| This Model is valid for Automotive grade 2 Temperature Range -40C<=Tc<=105C
| Valid for LPDDR4-4266 operation
| Part Number   VDD/VDDQ   Package   Architecture
| SCE11U32322EF-04ZA2   1.1 +0.07/-0.04  FBGA   1G   bit x 32 (200b,DDP,10x14.5x1.1)
| SCE11U16320EF-04ZA2   1.1 +0.07/-0.04  FBGA   512M bit x 32 (200b,SDP,10x14.5x1.1)
[IBIS Ver]  5.0
[File Name] usesnxx32fa2.ibs
[Date]   05/20/2025
[File Rev]  1.0
[Source] Simulation of a silicon level SPICE model
[Notes]  IBIS Characteristics for I/O Buffer
  IBIS Model Revision History: Rev 2.0:
  2026-03-27 - IBIS model file PN number change
[Disclaimer]  The IBIS models are for modeling purpose only and are subject to change without any notice. UniIC is not
  responsible for any problems the models may cause.
[Copyright] Copyright 2025 UniIC Semiconductors Corp. All rights reserved
|   Component SCE11U32322EF-04ZA2
[Component] SCE11U32322EF-04ZA2
[Manufacturer] UniIC Semiconductors Corp.
[Package]
|   typ   min   max
R_pkg   1104.5m   650.50m   1552.0m
L_pkg   2.074nH   1.252nH   2.895nH
C_pkg   0.931pF   0.710pF   1.151pF
[Pin] signal_name  model_name   R_pin   L_pin   C_pin
A1   DNU   NC
A2   DNU   NC
A3   VSS   GND
A4   VDD2   POWER
A5   ZQ0   NC
A8   NC   NC
A9   VDD2   POWER
A10   VSS   GND
A11   DNU   NC
A12   DNU   NC
B1   DNU   NC
B2   DQ0_A   DQ   847.00m   1.698nH   0.760pF
B3   VDDQ   POWER
B4   DQ7_A   DQ   926.00m   1.813nH   0.812pF
B5   VDDQ   POWER
B8   VDDQ   POWER
B9   DQ15_A   DQ   770.00m   1.540nH   0.721pF
B10   VDDQ   POWER
B11   DQ8_A   DQ   887.00m   1.780nH   0.770pF
B12   DNU   NC
C1   VSS   GND
C2   DQ1_A   DQ   875.00m   1.700nH   0.768pF
C3   DMI0_A   DQ   814.00m   1.560nH   0.737pF
C4   DQ6_A   DQ   807.82m   1.550nH   0.748pF
C5   VSS   GND
C8   VSS   GND
C9   DQ14_A   DQ   734.60m   1.445nH   0.710pF
C10   DMI1_A   DQ   797.00m   1.548nH   0.747pF
C11   DQ9_A   DQ   850.56m   1.652nH   0.773pF
C12   VSS   GND
D1   VDDQ   POWER
D2   VSS   GND
D3   DQS0_t_A   DQS   876.90m   1.604nH   0.763pF
D4   VSS   GND
D5   VDDQ   POWER
D8   VDDQ   POWER
D9   VSS   GND
D10   DQS1_t_A   DQS   887.69m   1.639nH   0.761pF
D11   VSS   GND
D12   VDDQ   POWER
E1   VSS   GND
E2   DQ2_A   DQ   762.89m   1.467nH   0.748pF
E3   DQS0_c_A   DQS   844.00m   1.542nH   0.754pF
E4   DQ5_A   DQ   703.98m   1.301nH   0.737pF
E5   VSS   GND
E8   VSS   GND
E9   DQ13_A   DQ   773.00m   1.436nH   0.777pF
E10   DQS1_c_A   DQS   883.30m   1.623nH   0.758pF
E11   DQ10_A   DQ   765.46m   1.468nH   0.760pF
E12   VSS   GND
F1   VDD1   POWER
F2   DQ3_A   DQ   779.40m   1.504nH   0.756pF
F3   VDDQ   POWER
F4   DQ4_A   DQ   716.48m   1.324nH   0.756pF
F5   VDD2   POWER
F8   VDD2   POWER
F9   DQ12_A   DQ   662.23m   1.252nH   0.714pF
F10   VDDQ   POWER
F11   DQ11_A   DQ   774.23m   1.506nH   0.768pF
F12   VDD1   POWER
G1   VSS   GND
G2   ODT_CA_A   ODTCA_INPUT   1136.0m   2.180nH   0.892pF
G3   VSS   GND
G4   VDD1   POWER
G5   VSS   GND
G8   VSS   GND
G9   VDD1   POWER
G10   VSS   GND
G11   NC   NC
G12   VSS   GND
H1   VDD2   POWER
H2   CA0_A   CA_INPUT   1398.8m   2.593nH   1.130pF
H3   CS1_A   CS_INPUT
H4   CS0_A   CS_INPUT
H5   VDD2   POWER
H8   VDD2   POWER
H9   CA2_A   CA_INPUT   1397.0m   2.554nH   1.150pF
H10   CA3_A   CA_INPUT   1148.0m   2.598nH   1.143pF
H11   CA4_A   CA_INPUT   1148.0m   2.709nH   1.153pF
H12   VDD2   POWER
J1   VSS   GND
J2   CA1_A   CA_INPUT   1453.0m   2.712nH   1.151pF
J3   VSS   GND
J4   CKE0_A   CKE_INPUT
J5   CKE1_A   CKE_INPUT
J8   CK_t_A   CLK_INPUT   1469.0m   2.704nH   1.078pF
J9   CK_c_A   CLK_INPUT   1486.0m   2.711nH   1.095pF
J10   VSS   GND
J11   CA5_A   CA_INPUT   1552.0m   2.895nH   1.206pF
J12   VSS   GND
K1   VDD2   POWER
K2   VSS   GND
K3   VDD2   POWER
K4   VSS   GND
K5   NC   NC
K8   NC   NC
K9   VSS   GND
K10   VDD2   POWER
K11   VSS   GND
K12   VDD2   POWER
N1   VDD2   POWER
N2   VSS   GND
N3   VDD2   POWER
N4   VSS   GND
N5   NC   NC
N8   NC   NC
N9   VSS   GND
N10   VDD2   POWER
N11   VSS   GND
N12   VDD2   POWER
P1   VSS   GND
P2   CA1_B   CA_INPUT   1442.0m   2.680nH   1.156pF
P3   VSS   GND
P4   CKE0_B   CKE_INPUT
P5   CKE1_B   CKE_INPUT
P8   CK_t_B   CLK_INPUT   1474.0m   2.686nH   1.065pF
P9   CK_c_B   CLK_INPUT   1481.0m   2.692nH   1.076pF
P10   VSS   GND
P11   CA5_B   CA_INPUT   1535.0m   2.859nH   1.204pF
P12   VSS   GND
R1   VDD2   POWER
R2   CA0_B   CA_INPUT   1435.0m   2.641nH   1.133pF
R3   CS1_B   CS_INPUT
R4   CS0_B   CS_INPUT
R5   VDD2   POWER
R8   VDD2   POWER
R9   CA2_B   CA_INPUT   1374.0m   2.528nH   1.124pF
R10   CA3_B   CA_INPUT   1373.0m   2.527nH   1.125pF
R11   CA4_B   CA_INPUT   1463.0m   2.722nH   1.149pF
R12   VDD2   POWER
T1   VSS   GND
T2   ODT_CA_B   ODTCA_INPUT   1146.0m   2.205nH   0.900pF
T3   VSS   GND
T4   VDD1   POWER
T5   VSS   GND
T8   VSS   GND
T9   VDD1   POWER
T10   VSS   GND
T11   RESET_n   NC
T12   VSS   GND
U1   VDD1   POWER
U2   DQ3_B   DQ   804.00m   1.559nH   0.763pF
U3   VDDQ   POWER
U4   DQ4_B   DQ   687.00m   1.284nH   0.716pF
U5   VDD2   POWER
U8   VDD2   POWER
U9   DQ12_B   DQ   672.30m   1.262nH   0.724pF
U10   VDDQ   POWER
U11   DQ11_B   DQ   777.17m   1.513nH   0.758pF
U12   VDD1   POWER
V1   VSS   GND
V2   DQ2_B   DQ   797.40m   1.539nH   0.769pF
V3   DQS0_c_B   DQS   861.50m   1.603nH   0.741pF
V4   DQ5_B   DQ   650.50m   1.233nH   0.701pF
V5   VSS   GND
V8   VSS   GND
V9   DQ13_B   DQ   648.00m   1.227nH   0.706pF
V10   DQS1_c_B   DQS   841.00m   1.538nH   0.744pF
V11   DQ10_B   DQ   771.40m   1.488nH   0.759pF
V12   VSS   GND
W1   VDDQ   POWER
W2   VSS   GND
W3   DQS0_t_B   DQS   839.00m   1.577nH   0.740pF
W4   VSS   GND
W5   VDDQ   POWER
W8   VDDQ   POWER
W9   VSS   GND
W10   DQS1_t_B   DQS   841.00m   1.547nH   0.733pF
W11   VSS   GND
W12   VDDQ   POWER
Y1   VSS   GND
Y2   DQ1_B   DQ   911.00m   1.744nH   0.787pF
Y3   DMI0_B   DQ   814.40m   1.570nH   0.726pF
Y4   DQ6_B   DQ   768.00m   1.499nH   0.718pF
Y5   VSS   GND
Y8   VSS   GND
Y9   DQ14_B   DQ   804.26m   1.578nH   0.754pF
Y10   DMI1_B   DQ   823.20m   1.578nH   0.761pF
Y11   DQ9_B   DQ   877.50m   1.697nH   0.780pF
Y12   VSS   GND
AA1   DNU   NC
AA2   DQ0_B   DQ   830.50m   1.680nH   0.752pF
AA3   VDDQ   POWER
AA4   DQ7_B   DQ   782.00m   1.584nH   0.730pF
AA5   VDDQ   POWER
AA8   VDDQ   POWER
AA9   DQ15_B   DQ   855.00m   1.687nH   0.761pF
AA10  VDDQ   POWER
AA11  DQ8_B   DQ   834.70m   1.680nH   0.751pF
AA12  DNU   NC
AB1   DNU   NC
AB2   DNU   NC
AB3   VSS   GND
AB4   VDD2   POWER
AB5   VSS   GND
AB8   VSS   GND
AB9   VDD2   POWER
AB10  VSS   GND
AB11  DNU   NC
AB12  DNU   NC
[Diff Pin]  inv_pin  vdiff   tdelay_typ   tdelay_min   tdelay_max
D3   E3   0.120V   0.000s   NA   NA
W3   V3   0.120V   0.000s   NA   NA
D10   E10   0.120V   0.000s   NA   NA
W10   V10   0.120V   0.000s   NA   NA
J8   J9   0.145V   0.000s   NA   NA
P8   P9   0.145V   0.000s   NA   NA
|   Component SCE11U16320EF-04ZA2
[Component] SCE11U16320EF-04ZA2
[Manufacturer] UniIC Semiconductors Corp.
[Package]
|   typ   min   max
R_pkg   1781.0m   683.00m   3340.0m
L_pkg   3.313nH   1.222nH   6.060nH
C_pkg   1.150pF   0.604pF   2.030pF
[Pin] signal_name  model_name   R_pin   L_pin   C_pin
A1   DNU   NC
A2   DNU   NC
A3   VSS   GND
A4   VDD2   POWER
A5   ZQ0   NC
A8   NC   NC
A9   VDD2   POWER
A10   VSS   GND
A11   DNU   NC
A12   DNU   NC
B1   DNU   NC
B2   DQ0_A   DQ   847.00m   1.698nH   0.760pF
B3   VDDQ   POWER
B4   DQ7_A   DQ   926.00m   1.813nH   0.812pF
B5   VDDQ   POWER
B8   VDDQ   POWER
B9   DQ15_A   DQ   770.00m   1.540nH   0.721pF
B10   VDDQ   POWER
B11   DQ8_A   DQ   887.00m   1.780nH   0.770pF
B12   DNU   NC
C1   VSS   GND
C2   DQ1_A   DQ   875.00m   1.700nH   0.768pF
C3   DMI0_A   DQ   814.00m   1.560nH   0.737pF
C4   DQ6_A   DQ   807.82m   1.550nH   0.748pF
C5   VSS   GND
C8   VSS   GND
C9   DQ14_A   DQ   734.60m   1.445nH   0.710pF
C10   DMI1_A   DQ   797.00m   1.548nH   0.747pF
C11   DQ9_A   DQ   850.56m   1.652nH   0.773pF
C12   VSS   GND
D1   VDDQ   POWER
D2   VSS   GND
D3   DQS0_t_A   DQS   876.90m   1.604nH   0.763pF
D4   VSS   GND
D5   VDDQ   POWER
D8   VDDQ   POWER
D9   VSS   GND
D10   DQS1_t_A   DQS   887.69m   1.639nH   0.761pF
D11   VSS   GND
D12   VDDQ   POWER
E1   VSS   GND
E2   DQ2_A   DQ   762.89m   1.467nH   0.748pF
E3   DQS0_c_A   DQS   844.00m   1.542nH   0.754pF
E4   DQ5_A   DQ   703.98m   1.301nH   0.737pF
E5   VSS   GND
E8   VSS   GND
E9   DQ13_A   DQ   773.00m   1.436nH   0.777pF
E10   DQS1_c_A   DQS   883.30m   1.623nH   0.758pF
E11   DQ10_A   DQ   765.46m   1.468nH   0.760pF
E12   VSS   GND
F1   VDD1   POWER
F2   DQ3_A   DQ   779.40m   1.504nH   0.756pF
F3   VDDQ   POWER
F4   DQ4_A   DQ   716.48m   1.324nH   0.756pF
F5   VDD2   POWER
F8   VDD2   POWER
F9   DQ12_A   DQ   662.23m   1.252nH   0.714pF
F10   VDDQ   POWER
F11   DQ11_A   DQ   774.23m   1.506nH   0.768pF
F12   VDD1   POWER
G1   VSS   GND
G2   ODT_CA_A   ODTCA_INPUT   1136.0m   2.180nH   0.892pF
G3   VSS   GND
G4   VDD1   POWER
G5   VSS   GND
G8   VSS   GND
G9   VDD1   POWER
G10   VSS   GND
G11   NC   NC
G12   VSS   GND
H1   VDD2   POWER
H2   CA0_A   CA_INPUT   1398.8m   2.593nH   1.13pF
H3   NC   NC
H4   CS0_A   CS_INPUT
H5   VDD2   POWER
H8   VDD2   POWER
H9   CA2_A   CA_INPUT   1397.0m   2.554nH   1.150pF
H10   CA3_A   CA_INPUT   1148.0m   2.598nH   1.143pF
H11   CA4_A   CA_INPUT   1148.0m   2.709nH   1.153pF
H12   VDD2   POWER
J1   VSS   GND
J2   CA1_A   CA_INPUT   1453.0m   2.712nH   1.151pF
J3   VSS   GND
J4   CKE0_A   CKE_INPUT
J5   NC   NC
J8   CK_t_A   CLK_INPUT   1469.0m   2.704nH   1.078pF
J9   CK_c_A   CLK_INPUT   1486.0m   2.711nH   1.095pF
J10   VSS   GND
J11   CA5_A   CA_INPUT   1552.0m   2.895nH   1.206pF
J12   VSS   GND
K1   VDD2   POWER
K2   VSS   GND
K3   VDD2   POWER
K4   VSS   GND
K5   NC   NC
K8   NC   NC
K9   VSS   GND
K10   VDD2   POWER
K11   VSS   GND
K12   VDD2   POWER
N1   VDD2   POWER
N2   VSS   GND
N3   VDD2   POWER
N4   VSS   GND
N5   NC   NC
N8   NC   NC
N9   VSS   GND
N10   VDD2   POWER
N11   VSS   GND
N12   VDD2   POWER
P1   VSS   GND
P2   CA1_B   CA_INPUT   1442.0m   2.680nH   1.156pF
P3   VSS   GND
P4   CKE0_B   CKE_INPUT
P5   NC   NC
P8   CK_t_B   CLK_INPUT   1474.0m   2.686nH   1.065pF
P9   CK_c_B   CLK_INPUT   1481.0m   2.692nH   1.076pF
P10   VSS   GND
P11   CA5_B   CA_INPUT   1535.0m   2.859nH   1.204pF
P12   VSS   GND
R1   VDD2   POWER
R2   CA0_B   CA_INPUT   1435.0m   2.641nH   1.133pF
R3   NC   NC
R4   CS0_B   CS_INPUT
R5   VDD2   POWER
R8   VDD2   POWER
R9   CA2_B   CA_INPUT   1374.0m   2.528nH   1.124pF
R10   CA3_B   CA_INPUT   1373.0m   2.527nH   1.125pF
R11   CA4_B   CA_INPUT   1463.0m   2.722nH   1.149pF
R12   VDD2   POWER
T1   VSS   GND
T2   ODT_CA_B   ODTCA_INPUT   1146.0m   2.205nH   0.900pF
T3   VSS   GND
T4   VDD1   POWER
T5   VSS   GND
T8   VSS   GND
T9   VDD1   POWER
T10   VSS   GND
T11   RESET_n   NC
T12   VSS   GND
U1   VDD1   POWER
U2   DQ3_B   DQ   804.00m   1.559nH   0.763pF
U3   VDDQ   POWER
U4   DQ4_B   DQ   687.00m   1.284nH   0.716pF
U5   VDD2   POWER
U8   VDD2   POWER
U9   DQ12_B   DQ   672.30m   1.262nH   0.724pF
U10   VDDQ   POWER
U11   DQ11_B   DQ   777.17m   1.513nH   0.758pF
U12   VDD1   POWER
V1   VSS   GND
V2   DQ2_B   DQ   797.40m   1.539nH   0.769pF
V3   DQS0_c_B   DQS   861.50m   1.603nH   0.741pF
V4   DQ5_B   DQ   650.50m   1.233nH   0.701pF
V5   VSS   GND
V8   VSS   GND
V9   DQ13_B   DQ   648.00m   1.227nH   0.706pF
V10   DQS1_c_B   DQS   841.00m   1.538nH   0.744pF
V11   DQ10_B   DQ   771.40m   1.488nH   0.759pF
V12   VSS   GND
W1   VDDQ   POWER
W2   VSS   GND
W3   DQS0_t_B   DQS   839.00m   1.577nH   0.740pF
W4   VSS   GND
W5   VDDQ   POWER
W8   VDDQ   POWER
W9   VSS   GND
W10   DQS1_t_B   DQS   841.00m   1.547nH   0.733pF
W11   VSS   GND
W12   VDDQ   POWER
Y1   VSS   GND
Y2   DQ1_B   DQ   911.00m   1.744nH   0.787pF
Y3   DMI0_B   DQ   814.40m   1.570nH   0.726pF
Y4   DQ6_B   DQ   768.00m   1.499nH   0.718pF
Y5   VSS   GND
Y8   VSS   GND
Y9   DQ14_B   DQ   804.26m   1.578nH   0.754pF
Y10   DMI1_B   DQ   823.20m   1.578nH   0.761pF
Y11   DQ9_B   DQ   877.50m   1.697nH   0.780pF
Y12   VSS   GND
AA1   DNU   NC
AA2   DQ0_B   DQ   830.50m   1.680nH   0.752pF
AA3   VDDQ   POWER
AA4   DQ7_B   DQ   782.00m   1.584nH   0.730pF
AA5   VDDQ   POWER
AA8   VDDQ   POWER
AA9   DQ15_B   DQ   855.00m   1.687nH   0.761pF
AA10  VDDQ   POWER
AA11  DQ8_B   DQ   834.70m   1.680nH   0.751pF
AA12  DNU   NC
AB1   DNU   NC
AB2   DNU   NC
AB3   VSS   GND
AB4   VDD2   POWER
AB5   VSS   GND
AB8   VSS   GND
AB9   VDD2   POWER
AB10  VSS   GND
AB11  DNU   NC
AB12  DNU   NC
[Diff Pin]  inv_pin  vdiff   tdelay_typ   tdelay_min   tdelay_max
D3   E3   0.120V   0.000s   NA   NA
W3   V3   0.120V   0.000s   NA   NA
D10   E10   0.120V   0.000s   NA   NA
W10   V10   0.120V   0.000s   NA   NA
J8   J9   0.145V   0.000s   NA   NA
P8   P9   0.145V   0.000s   NA   NA
|   Model Selector
[Model Selector] DQ
| Data I/O models
DQ_PD40_SOC-ODT40_VOH30_4266   40 Ohm Pulldown, 40 Ohm System ODT Setting, VOH=VDDQ/3.0, 3200-4266Mbps
DQ_PD40_SOC-ODT48_VOH30_4266   40 Ohm Pulldown, 48 Ohm System ODT Setting, VOH=VDDQ/3.0, 3200-4266Mbps
DQ_PD40_SOC-ODT60_VOH30_4266   40 Ohm Pulldown, 60 Ohm System ODT Setting, VOH=VDDQ/3.0, 3200-4266Mbps
DQ_PD40_SOC-ODT80_VOH30_4266   40 Ohm Pulldown, 80 Ohm System ODT Setting, VOH=VDDQ/3.0, 3200-4266Mbps
DQ_PD40_SOC-ODT120_VOH30_4266   40 Ohm Pulldown, 120 Ohm System ODT Setting, VOH=VDDQ/3.0, 3200-4266Mbps
DQ_PD40_SOC-ODT240_VOH30_4266   40 Ohm Pulldown, 240 Ohm System ODT Setting, VOH=VDDQ/3.0, 3200-4266Mbps
DQ_PD40_SOC-ODTDIS_VOH30_4266   40 Ohm Pulldown, SOC ODT disabled setting, VOH=VDDQ/3.0 cal. point, 3200-4266Mbps
DQ_PD40_SOC-ODT80_VOH25_4266   40 Ohm Pulldown, 80 Ohm System ODT Setting, VOH=VDDQ/2.5, 3200-4266Mbps
DQ_PD40_SOC-ODT120_VOH25_4266   40 Ohm Pulldown, 120 Ohm System ODT Setting, VOH=VDDQ/2.5, 3200-4266Mbps
DQ_PD40_SOC-ODT240_VOH25_4266   40 Ohm Pulldown, 240 Ohm System ODT Setting, VOH=VDDQ/2.5, 3200-4266Mbps
DQ_PD40_SOC-ODTDIS_VOH25_4266   40 Ohm Pulldown, SOC ODT disabled setting, VOH=VDDQ/2.5 cal. point, 3200-4266Mbps
DQ_PD48_SOC-ODT40_VOH30_4266   48 Ohm Pulldown, 40 Ohm System ODT Setting, VOH=VDDQ/3.0, 3200-4266Mbps
DQ_PD48_SOC-ODT48_VOH30_4266   48 Ohm Pulldown, 48 Ohm System ODT Setting, VOH=VDDQ/3.0, 3200-4266Mbps
DQ_PD48_SOC-ODT60_VOH30_4266   48 Ohm Pulldown, 60 Ohm System ODT Setting, VOH=VDDQ/3.0, 3200-4266Mbps
DQ_PD48_SOC-ODT80_VOH30_4266   48 Ohm Pulldown, 80 Ohm System ODT Setting, VOH=VDDQ/3.0, 3200-4266Mbps
DQ_PD48_SOC-ODT120_VOH30_4266   48 Ohm Pulldown, 120 Ohm System ODT Setting, VOH=VDDQ/3.0, 3200-4266Mbps
DQ_PD48_SOC-ODT240_VOH30_4266   48 Ohm Pulldown, 240 Ohm System ODT Setting, VOH=VDDQ/3.0, 3200-4266Mbps
DQ_PD48_SOC-ODTDIS_VOH30_4266   48 Ohm Pulldown, SOC ODT disabled setting, VOH=VDDQ/3.0 cal. point, 3200-4266Mbps
DQ_PD48_SOC-ODT80_VOH25_4266   48 Ohm Pulldown, 80 Ohm System ODT Setting, VOH=VDDQ/2.5, 3200-4266Mbps
DQ_PD48_SOC-ODT120_VOH25_4266   48 Ohm Pulldown, 120 Ohm System ODT Setting, VOH=VDDQ/2.5, 3200-4266Mbps
DQ_PD48_SOC-ODT240_VOH25_4266   48 Ohm Pulldown, 240 Ohm System ODT Setting, VOH=VDDQ/2.5, 3200-4266Mbps
DQ_PD48_SOC-ODTDIS_VOH25_4266   48 Ohm Pulldown, SOC ODT disabled setting, VOH=VDDQ/2.5 cal. point, 3200-4266Mbps
DQ_PD60_SOC-ODT40_VOH30_4266   60 Ohm Pulldown, 40 Ohm System ODT Setting, VOH=VDDQ/3.0, 3200-4266Mbps
DQ_PD60_SOC-ODT48_VOH30_4266   60 Ohm Pulldown, 48 Ohm System ODT Setting, VOH=VDDQ/3.0, 3200-4266Mbps
DQ_PD60_SOC-ODT60_VOH30_4266   60 Ohm Pulldown, 60 Ohm System ODT Setting, VOH=VDDQ/3.0, 3200-4266Mbps
DQ_PD60_SOC-ODT80_VOH30_4266   60 Ohm Pulldown, 80 Ohm System ODT Setting, VOH=VDDQ/3.0, 3200-4266Mbps
DQ_PD60_SOC-ODT120_VOH30_4266   60 Ohm Pulldown, 120 Ohm System ODT Setting, VOH=VDDQ/3.0, 3200-4266Mbps
DQ_PD60_SOC-ODT240_VOH30_4266   60 Ohm Pulldown, 240 Ohm System ODT Setting, VOH=VDDQ/3.0, 3200-4266Mbps
DQ_PD60_SOC-ODTDIS_VOH30_4266   60 Ohm Pulldown, SOC ODT disabled setting, VOH=VDDQ/3.0 cal. point, 3200-4266Mbps
DQ_PD60_SOC-ODT80_VOH25_4266   60 Ohm Pulldown, 80 Ohm System ODT Setting, VOH=VDDQ/2.5, 3200-4266Mbps
DQ_PD60_SOC-ODT120_VOH25_4266   60 Ohm Pulldown, 120 Ohm System ODT Setting, VOH=VDDQ/2.5, 3200-4266Mbps
DQ_PD60_SOC-ODT240_VOH25_4266   60 Ohm Pulldown, 240 Ohm System ODT Setting, VOH=VDDQ/2.5, 3200-4266Mbps
DQ_PD60_SOC-ODTDIS_VOH25_4266   60 Ohm Pulldown, SOC ODT disabled setting, VOH=VDDQ/2.5 cal. point, 3200-4266Mbps
DQ_PD80_SOC-ODT40_VOH30_4266   80 Ohm Pulldown, 40 Ohm System ODT Setting, VOH=VDDQ/3.0, 3200-4266Mbps
DQ_PD80_SOC-ODT48_VOH30_4266   80 Ohm Pulldown, 48 Ohm System ODT Setting, VOH=VDDQ/3.0, 3200-4266Mbps
DQ_PD80_SOC-ODT60_VOH30_4266   80 Ohm Pulldown, 60 Ohm System ODT Setting, VOH=VDDQ/3.0, 3200-4266Mbps
DQ_PD80_SOC-ODT80_VOH30_4266   80 Ohm Pulldown, 80 Ohm System ODT Setting, VOH=VDDQ/3.0, 3200-4266Mbps
DQ_PD80_SOC-ODT120_VOH30_4266   80 Ohm Pulldown, 120 Ohm System ODT Setting, VOH=VDDQ/3.0, 3200-4266Mbps
DQ_PD80_SOC-ODT240_VOH30_4266   80 Ohm Pulldown, 240 Ohm System ODT Setting, VOH=VDDQ/3.0, 3200-4266Mbps
DQ_PD80_SOC-ODTDIS_VOH30_4266   80 Ohm Pulldown, SOC ODT disabled setting, VOH=VDDQ/3.0 cal. point, 3200-4266Mbps
DQ_PD80_SOC-ODT80_VOH25_4266   80 Ohm Pulldown, 80 Ohm System ODT Setting, VOH=VDDQ/2.5, 3200-4266Mbps
DQ_PD80_SOC-ODT120_VOH25_4266   80 Ohm Pulldown, 120 Ohm System ODT Setting, VOH=VDDQ/2.5, 3200-4266Mbps
DQ_PD80_SOC-ODT240_VOH25_4266   80 Ohm Pulldown, 240 Ohm System ODT Setting, VOH=VDDQ/2.5, 3200-4266Mbps
DQ_PD80_SOC-ODTDIS_VOH25_4266   80 Ohm Pulldown, SOC ODT disabled setting, VOH=VDDQ/2.5 cal. point, 3200-4266Mbps
DQ_PD120_SOC-ODT40_VOH30_4266   120 Ohm Pulldown, 40 Ohm System ODT Setting, VOH=VDDQ/3.0, 3200-4266Mbps
DQ_PD120_SOC-ODT48_VOH30_4266   120 Ohm Pulldown, 48 Ohm System ODT Setting, VOH=VDDQ/3.0, 3200-4266Mbps
DQ_PD120_SOC-ODT60_VOH30_4266   120 Ohm Pulldown, 60 Ohm System ODT Setting, VOH=VDDQ/3.0, 3200-4266Mbps
DQ_PD120_SOC-ODT80_VOH30_4266   120 Ohm Pulldown, 80 Ohm System ODT Setting, VOH=VDDQ/3.0, 3200-4266Mbps
DQ_PD120_SOC-ODT120_VOH30_4266  120 Ohm Pulldown, 120 Ohm System ODT Setting, VOH=VDDQ/3.0, 3200-4266Mbps
DQ_PD120_SOC-ODT240_VOH30_4266  120 Ohm Pulldown, 240 Ohm System ODT Setting, VOH=VDDQ/3.0, 3200-4266Mbps
DQ_PD120_SOC-ODTDIS_VOH30_4266  120 Ohm Pulldown, SOC ODT disabled setting, VOH=VDDQ/3.0 cal. point, 3200-4266Mbps
DQ_PD120_SOC-ODT80_VOH25_4266   120 Ohm Pulldown, 80 Ohm System ODT Setting, VOH=VDDQ/2.5, 3200-4266Mbps
DQ_PD120_SOC-ODT120_VOH25_4266  120 Ohm Pulldown, 120 Ohm System ODT Setting, VOH=VDDQ/2.5, 3200-4266Mbps
DQ_PD120_SOC-ODT240_VOH25_4266  120 Ohm Pulldown, 240 Ohm System ODT Setting, VOH=VDDQ/2.5, 3200-4266Mbps
DQ_PD120_SOC-ODTDIS_VOH25_4266  120 Ohm Pulldown, SOC ODT disabled setting, VOH=VDDQ/2.5 cal. point, 3200-4266Mbps
DQ_PD240_SOC-ODT40_VOH30_4266   240 Ohm Pulldown, 40 Ohm System ODT Setting, VOH=VDDQ/3.0, 3200-4266Mbps
DQ_PD240_SOC-ODT48_VOH30_4266   240 Ohm Pulldown, 48 Ohm System ODT Setting, VOH=VDDQ/3.0, 3200-4266Mbps
DQ_PD240_SOC-ODT60_VOH30_4266   240 Ohm Pulldown, 60 Ohm System ODT Setting, VOH=VDDQ/3.0, 3200-4266Mbps
DQ_PD240_SOC-ODT80_VOH30_4266   240 Ohm Pulldown, 80 Ohm System ODT Setting, VOH=VDDQ/3.0, 3200-4266Mbps
DQ_PD240_SOC-ODT120_VOH30_4266  240 Ohm Pulldown, 120 Ohm System ODT Setting, VOH=VDDQ/3.0, 3200-4266Mbps
DQ_PD240_SOC-ODT240_VOH30_4266  240 Ohm Pulldown, 240 Ohm System ODT Setting, VOH=VDDQ/3.0, 3200-4266Mbps
DQ_PD240_SOC-ODTDIS_VOH30_4266  240 Ohm Pulldown, SOC ODT disabled setting, VOH=VDDQ/3.0 cal. point, 3200-4266Mbps
DQ_PD240_SOC-ODT80_VOH25_4266   240 Ohm Pulldown, 80 Ohm System ODT Setting, VOH=VDDQ/2.5, 3200-4266Mbps
DQ_PD240_SOC-ODT120_VOH25_4266  240 Ohm Pulldown, 120 Ohm System ODT Setting, VOH=VDDQ/2.5, 3200-4266Mbps
DQ_PD240_SOC-ODT240_VOH25_4266  240 Ohm Pulldown, 240 Ohm System ODT Setting, VOH=VDDQ/2.5, 3200-4266Mbps
DQ_PD240_SOC-ODTDIS_VOH25_4266  240 Ohm Pulldown, SOC ODT disabled setting, VOH=VDDQ/2.5 cal. point, 3200-4266Mbps
DQ_IN_ODTOFF_4266   with no ODT, 3200-4266Mbps
DQ_IN_ODT40_4266   with 40ohm ODT, 3200-4266Mbps
DQ_IN_ODT48_4266   with 48ohm ODT, 3200-4266Mbps
DQ_IN_ODT60_4266   with 60ohm ODT, 3200-4266Mbps
DQ_IN_ODT80_4266   with 80ohm ODT, 3200-4266Mbps
DQ_IN_ODT120_4266   with 120ohm ODT, 3200-4266Mbps
DQ_IN_ODT240_4266   with 240ohm ODT, 3200-4266Mbps
[Model Selector] DQS
| Data Strobe I/O models
DQS_PD40_SOC-ODT40_VOH30_4266   40 Ohm Pulldown, 40 Ohm System ODT Setting, VOH=VDDQ/3.0, 3200-4266Mbps
DQS_PD40_SOC-ODT48_VOH30_4266   40 Ohm Pulldown, 48 Ohm System ODT Setting, VOH=VDDQ/3.0, 3200-4266Mbps
DQS_PD40_SOC-ODT60_VOH30_4266   40 Ohm Pulldown, 60 Ohm System ODT Setting, VOH=VDDQ/3.0, 3200-4266Mbps
DQS_PD40_SOC-ODT80_VOH30_4266   40 Ohm Pulldown, 80 Ohm System ODT Setting, VOH=VDDQ/3.0, 3200-4266Mbps
DQS_PD40_SOC-ODT120_VOH30_4266  40 Ohm Pulldown, 120 Ohm System ODT Setting, VOH=VDDQ/3.0, 3200-4266Mbps
DQS_PD40_SOC-ODT240_VOH30_4266  40 Ohm Pulldown, 240 Ohm System ODT Setting, VOH=VDDQ/3.0, 3200-4266Mbps
DQS_PD40_SOC-ODTDIS_VOH30_4266  40 Ohm Pulldown, SOC ODT disabled setting, VOH=VDDQ/3.0 cal. point, 3200-4266Mbps
DQS_PD40_SOC-ODT80_VOH25_4266   40 Ohm Pulldown, 80 Ohm System ODT Setting, VOH=VDDQ/2.5, 3200-4266Mbps
DQS_PD40_SOC-ODT120_VOH25_4266  40 Ohm Pulldown, 120 Ohm System ODT Setting, VOH=VDDQ/2.5, 3200-4266Mbps
DQS_PD40_SOC-ODT240_VOH25_4266  40 Ohm Pulldown, 240 Ohm System ODT Setting, VOH=VDDQ/2.5, 3200-4266Mbps
DQS_PD40_SOC-ODTDIS_VOH25_4266  40 Ohm Pulldown, SOC ODT disabled setting, VOH=VDDQ/2.5 cal. point, 3200-4266Mbps
DQS_PD48_SOC-ODT40_VOH30_4266   48 Ohm Pulldown, 40 Ohm System ODT Setting, VOH=VDDQ/3.0, 3200-4266Mbps
DQS_PD48_SOC-ODT48_VOH30_4266   48 Ohm Pulldown, 48 Ohm System ODT Setting, VOH=VDDQ/3.0, 3200-4266Mbps
DQS_PD48_SOC-ODT60_VOH30_4266   48 Ohm Pulldown, 60 Ohm System ODT Setting, VOH=VDDQ/3.0, 3200-4266Mbps
DQS_PD48_SOC-ODT80_VOH30_4266   48 Ohm Pulldown, 80 Ohm System ODT Setting, VOH=VDDQ/3.0, 3200-4266Mbps
DQS_PD48_SOC-ODT120_VOH30_4266  48 Ohm Pulldown, 120 Ohm System ODT Setting, VOH=VDDQ/3.0, 3200-4266Mbps
DQS_PD48_SOC-ODT240_VOH30_4266  48 Ohm Pulldown, 240 Ohm System ODT Setting, VOH=VDDQ/3.0, 3200-4266Mbps
DQS_PD48_SOC-ODTDIS_VOH30_4266  48 Ohm Pulldown, SOC ODT disabled setting, VOH=VDDQ/3.0 cal. point, 3200-4266Mbps
DQS_PD48_SOC-ODT80_VOH25_4266   48 Ohm Pulldown, 80 Ohm System ODT Setting, VOH=VDDQ/2.5, 3200-4266Mbps
DQS_PD48_SOC-ODT120_VOH25_4266  48 Ohm Pulldown, 120 Ohm System ODT Setting, VOH=VDDQ/2.5, 3200-4266Mbps
DQS_PD48_SOC-ODT240_VOH25_4266  48 Ohm Pulldown, 240 Ohm System ODT Setting, VOH=VDDQ/2.5, 3200-4266Mbps
DQS_PD48_SOC-ODTDIS_VOH25_4266  48 Ohm Pulldown, SOC ODT disabled setting, VOH=VDDQ/2.5 cal. point, 3200-4266Mbps
DQS_PD60_SOC-ODT40_VOH30_4266   60 Ohm Pulldown, 40 Ohm System ODT Setting, VOH=VDDQ/3.0, 3200-4266Mbps
DQS_PD60_SOC-ODT48_VOH30_4266   60 Ohm Pulldown, 48 Ohm System ODT Setting, VOH=VDDQ/3.0, 3200-4266Mbps
DQS_PD60_SOC-ODT60_VOH30_4266   60 Ohm Pulldown, 60 Ohm System ODT Setting, VOH=VDDQ/3.0, 3200-4266Mbps
DQS_PD60_SOC-ODT80_VOH30_4266   60 Ohm Pulldown, 80 Ohm System ODT Setting, VOH=VDDQ/3.0, 3200-4266Mbps
DQS_PD60_SOC-ODT120_VOH30_4266  60 Ohm Pulldown, 120 Ohm System ODT Setting, VOH=VDDQ/3.0, 3200-4266Mbps
DQS_PD60_SOC-ODT240_VOH30_4266  60 Ohm Pulldown, 240 Ohm System ODT Setting, VOH=VDDQ/3.0, 3200-4266Mbps
DQS_PD60_SOC-ODTDIS_VOH30_4266  60 Ohm Pulldown, SOC ODT disabled setting, VOH=VDDQ/3.0 cal. point, 3200-4266Mbps
DQS_PD60_SOC-ODT80_VOH25_4266   60 Ohm Pulldown, 80 Ohm System ODT Setting, VOH=VDDQ/2.5, 3200-4266Mbps
DQS_PD60_SOC-ODT120_VOH25_4266  60 Ohm Pulldown, 120 Ohm System ODT Setting, VOH=VDDQ/2.5, 3200-4266Mbps
DQS_PD60_SOC-ODT240_VOH25_4266  60 Ohm Pulldown, 240 Ohm System ODT Setting, VOH=VDDQ/2.5, 3200-4266Mbps
DQS_PD60_SOC-ODTDIS_VOH25_4266  60 Ohm Pulldown, SOC ODT disabled setting, VOH=VDDQ/2.5 cal. point, 3200-4266Mbps
DQS_PD80_SOC-ODT40_VOH30_4266   80 Ohm Pulldown, 40 Ohm System ODT Setting, VOH=VDDQ/3.0, 3200-4266Mbps
DQS_PD80_SOC-ODT48_VOH30_4266   80 Ohm Pulldown, 48 Ohm System ODT Setting, VOH=VDDQ/3.0, 3200-4266Mbps
DQS_PD80_SOC-ODT60_VOH30_4266   80 Ohm Pulldown, 60 Ohm System ODT Setting, VOH=VDDQ/3.0, 3200-4266Mbps
DQS_PD80_SOC-ODT80_VOH30_4266   80 Ohm Pulldown, 80 Ohm System ODT Setting, VOH=VDDQ/3.0, 3200-4266Mbps
DQS_PD80_SOC-ODT120_VOH30_4266  80 Ohm Pulldown, 120 Ohm System ODT Setting, VOH=VDDQ/3.0, 3200-4266Mbps
DQS_PD80_SOC-ODT240_VOH30_4266  80 Ohm Pulldown, 240 Ohm System ODT Setting, VOH=VDDQ/3.0, 3200-4266Mbps
DQS_PD80_SOC-ODTDIS_VOH30_4266  80 Ohm Pulldown, SOC ODT disabled setting, VOH=VDDQ/3.0 cal. point, 3200-4266Mbps
DQS_PD80_SOC-ODT80_VOH25_4266   80 Ohm Pulldown, 80 Ohm System ODT Setting, VOH=VDDQ/2.5, 3200-4266Mbps
DQS_PD80_SOC-ODT120_VOH25_4266  80 Ohm Pulldown, 120 Ohm System ODT Setting, VOH=VDDQ/2.5, 3200-4266Mbps
DQS_PD80_SOC-ODT240_VOH25_4266  80 Ohm Pulldown, 240 Ohm System ODT Setting, VOH=VDDQ/2.5, 3200-4266Mbps
DQS_PD80_SOC-ODTDIS_VOH25_4266  80 Ohm Pulldown, SOC ODT disabled setting, VOH=VDDQ/2.5 cal. point, 3200-4266Mbps
DQS_PD120_SOC-ODT40_VOH30_4266  120 Ohm Pulldown, 40 Ohm System ODT Setting, VOH=VDDQ/3.0, 3200-4266Mbps
DQS_PD120_SOC-ODT48_VOH30_4266  120 Ohm Pulldown, 48 Ohm System ODT Setting, VOH=VDDQ/3.0, 3200-4266Mbps
DQS_PD120_SOC-ODT60_VOH30_4266  120 Ohm Pulldown, 60 Ohm System ODT Setting, VOH=VDDQ/3.0, 3200-4266Mbps
DQS_PD120_SOC-ODT80_VOH30_4266  120 Ohm Pulldown, 80 Ohm System ODT Setting, VOH=VDDQ/3.0, 3200-4266Mbps
DQS_PD120_SOC-ODT120_VOH30_4266 120 Ohm Pulldown, 120 Ohm System ODT Setting, VOH=VDDQ/3.0, 3200-4266Mbps
DQS_PD120_SOC-ODT240_VOH30_4266 120 Ohm Pulldown, 240 Ohm System ODT Setting, VOH=VDDQ/3.0, 3200-4266Mbps
DQS_PD120_SOC-ODTDIS_VOH30_4266 120 Ohm Pulldown, SOC ODT disabled setting, VOH=VDDQ/3.0 cal. point, 3200-4266Mbps
DQS_PD120_SOC-ODT80_VOH25_4266  120 Ohm Pulldown, 80 Ohm System ODT Setting, VOH=VDDQ/2.5, 3200-4266Mbps
DQS_PD120_SOC-ODT120_VOH25_4266 120 Ohm Pulldown, 120 Ohm System ODT Setting, VOH=VDDQ/2.5, 3200-4266Mbps
DQS_PD120_SOC-ODT240_VOH25_4266 120 Ohm Pulldown, 240 Ohm System ODT Setting, VOH=VDDQ/2.5, 3200-4266Mbps
DQS_PD120_SOC-ODTDIS_VOH25_4266 120 Ohm Pulldown, SOC ODT disabled setting, VOH=VDDQ/2.5 cal. point, 3200-4266Mbps
DQS_PD240_SOC-ODT40_VOH30_4266  240 Ohm Pulldown, 40 Ohm System ODT Setting, VOH=VDDQ/3.0, 3200-4266Mbps
DQS_PD240_SOC-ODT48_VOH30_4266  240 Ohm Pulldown, 48 Ohm System ODT Setting, VOH=VDDQ/3.0, 3200-4266Mbps
DQS_PD240_SOC-ODT60_VOH30_4266  240 Ohm Pulldown, 60 Ohm System ODT Setting, VOH=VDDQ/3.0, 3200-4266Mbps
DQS_PD240_SOC-ODT80_VOH30_4266  240 Ohm Pulldown, 80 Ohm System ODT Setting, VOH=VDDQ/3.0, 3200-4266Mbps
DQS_PD240_SOC-ODT120_VOH30_4266 240 Ohm Pulldown, 120 Ohm System ODT Setting, VOH=VDDQ/3.0, 3200-4266Mbps
DQS_PD240_SOC-ODT240_VOH30_4266 240 Ohm Pulldown, 240 Ohm System ODT Setting, VOH=VDDQ/3.0, 3200-4266Mbps
DQS_PD240_SOC-ODTDIS_VOH30_4266 240 Ohm Pulldown, SOC ODT disabled setting, VOH=VDDQ/3.0 cal. point, 3200-4266Mbps
DQS_PD240_SOC-ODT80_VOH25_4266  240 Ohm Pulldown, 80 Ohm System ODT Setting, VOH=VDDQ/2.5, 3200-4266Mbps
DQS_PD240_SOC-ODT120_VOH25_4266 240 Ohm Pulldown, 120 Ohm System ODT Setting, VOH=VDDQ/2.5, 3200-4266Mbps
DQS_PD240_SOC-ODT240_VOH25_4266 240 Ohm Pulldown, 240 Ohm System ODT Setting, VOH=VDDQ/2.5, 3200-4266Mbps
DQS_PD240_SOC-ODTDIS_VOH25_4266 240 Ohm Pulldown, SOC ODT disabled setting, VOH=VDDQ/2.5 cal. point, 3200-4266Mbps
DQS_IN_ODTOFF_4266   with no ODT, 3200-4266Mbps
DQS_IN_ODT40_4266   with 40ohm ODT, 3200-4266Mbps
DQS_IN_ODT48_4266   with 48ohm ODT, 3200-4266Mbps
DQS_IN_ODT60_4266   with 60ohm ODT, 3200-4266Mbps
DQS_IN_ODT80_4266   with 80ohm ODT, 3200-4266Mbps
DQS_IN_ODT120_4266   with 120ohm ODT, 3200-4266Mbps
DQS_IN_ODT240_4266   with 240ohm ODT, 3200-4266Mbps
[Model Selector] CA_INPUT
| CA Input models
CA_INPUT_ODTOFF_4266   with no ODT, 3200-4266Mbps
CA_INPUT_ODT40_4266   with 40ohm ODT, 3200-4266Mbps
CA_INPUT_ODT48_4266   with 48ohm ODT, 3200-4266Mbps
CA_INPUT_ODT60_4266   with 60ohm ODT, 3200-4266Mbps
CA_INPUT_ODT80_4266   with 80ohm ODT, 3200-4266Mbps
CA_INPUT_ODT120_4266   with 120ohm ODT, 3200-4266Mbps
CA_INPUT_ODT240_4266   with 240ohm ODT, 3200-4266Mbps
[Model Selector] CS_INPUT
| CS Input models
CS_INPUT_ODTOFF_4266   with no ODT, 3200-4266Mbps
CS_INPUT_ODT40_4266   with 40ohm ODT, 3200-4266Mbps
CS_INPUT_ODT48_4266   with 48ohm ODT, 3200-4266Mbps
CS_INPUT_ODT60_4266   with 60ohm ODT, 3200-4266Mbps
CS_INPUT_ODT80_4266   with 80ohm ODT, 3200-4266Mbps
CS_INPUT_ODT120_4266   with 120ohm ODT, 3200-4266Mbps
CS_INPUT_ODT240_4266   with 240ohm ODT, 3200-4266Mbps
[Model Selector] CLK_INPUT
| Clock Input models
CLK_INPUT_ODTOFF_4266   with no ODT, 3200-4266Mbps
CLK_INPUT_ODT40_4266   with 40ohm ODT, 3200-4266Mbps
CLK_INPUT_ODT48_4266   with 48ohm ODT, 3200-4266Mbps
CLK_INPUT_ODT60_4266   with 60ohm ODT, 3200-4266Mbps
CLK_INPUT_ODT80_4266   with 80ohm ODT, 3200-4266Mbps
CLK_INPUT_ODT120_4266   with 120ohm ODT, 3200-4266Mbps
CLK_INPUT_ODT240_4266   with 240ohm ODT, 3200-4266Mbps
| Models and submodels in the file (175): DQ_PD40_SOC-ODT40_VOH30_4266 (I/O), DQ_PD40_SOC-ODT48_VOH30_4266 (I/O), DQ_PD40_SOC-ODT60_VOH30_4266 (I/O), DQ_PD40_SOC-ODT80_VOH30_4266 (I/O), DQ_PD40_SOC-ODT120_VOH30_4266 (I/O), DQ_PD40_SOC-ODT240_VOH30_4266 (I/O), DQ_PD40_SOC-ODTDIS_VOH30_4266 (I/O), DQ_PD40_SOC-ODT80_VOH25_4266 (I/O), DQ_PD40_SOC-ODT120_VOH25_4266 (I/O), DQ_PD40_SOC-ODT240_VOH25_4266 (I/O), DQ_PD40_SOC-ODTDIS_VOH25_4266 (I/O), DQ_PD48_SOC-ODT40_VOH30_4266 (I/O), DQ_PD48_SOC-ODT48_VOH30_4266 (I/O), DQ_PD48_SOC-ODT60_VOH30_4266 (I/O), DQ_PD48_SOC-ODT80_VOH30_4266 (I/O), DQ_PD48_SOC-ODT120_VOH30_4266 (I/O), DQ_PD48_SOC-ODT240_VOH30_4266 (I/O), DQ_PD48_SOC-ODTDIS_VOH30_4266 (I/O), DQ_PD48_SOC-ODT80_VOH25_4266 (I/O), DQ_PD48_SOC-ODT120_VOH25_4266 (I/O), DQ_PD48_SOC-ODT240_VOH25_4266 (I/O), DQ_PD48_SOC-ODTDIS_VOH25_4266 (I/O), DQ_PD60_SOC-ODT40_VOH30_4266 (I/O), DQ_PD60_SOC-ODT48_VOH30_4266 (I/O), DQ_PD60_SOC-ODT60_VOH30_4266 (I/O), DQ_PD60_SOC-ODT80_VOH30_4266 (I/O), DQ_PD60_SOC-ODT120_VOH30_4266 (I/O), DQ_PD60_SOC-ODT240_VOH30_4266 (I/O), DQ_PD60_SOC-ODTDIS_VOH30_4266 (I/O), DQ_PD60_SOC-ODT80_VOH25_4266 (I/O), DQ_PD60_SOC-ODT120_VOH25_4266 (I/O), DQ_PD60_SOC-ODT240_VOH25_4266 (I/O), DQ_PD60_SOC-ODTDIS_VOH25_4266 (I/O), DQ_PD80_SOC-ODT40_VOH30_4266 (I/O), DQ_PD80_SOC-ODT48_VOH30_4266 (I/O), DQ_PD80_SOC-ODT60_VOH30_4266 (I/O), DQ_PD80_SOC-ODT80_VOH30_4266 (I/O), DQ_PD80_SOC-ODT120_VOH30_4266 (I/O), DQ_PD80_SOC-ODT240_VOH30_4266 (I/O), DQ_PD80_SOC-ODTDIS_VOH30_4266 (I/O), DQ_PD80_SOC-ODT80_VOH25_4266 (I/O), DQ_PD80_SOC-ODT120_VOH25_4266 (I/O), DQ_PD80_SOC-ODT240_VOH25_4266 (I/O), DQ_PD80_SOC-ODTDIS_VOH25_4266 (I/O), DQ_PD120_SOC-ODT40_VOH30_4266 (I/O), DQ_PD120_SOC-ODT48_VOH30_4266 (I/O), DQ_PD120_SOC-ODT60_VOH30_4266 (I/O), DQ_PD120_SOC-ODT80_VOH30_4266 (I/O), DQ_PD120_SOC-ODT120_VOH30_4266 (I/O), DQ_PD120_SOC-ODT240_VOH30_4266 (I/O), DQ_PD120_SOC-ODTDIS_VOH30_4266 (I/O), DQ_PD120_SOC-ODT80_VOH25_4266 (I/O), DQ_PD120_SOC-ODT120_VOH25_4266 (I/O), DQ_PD120_SOC-ODT240_VOH25_4266 (I/O), DQ_PD120_SOC-ODTDIS_VOH25_4266 (I/O), DQ_PD240_SOC-ODT40_VOH30_4266 (I/O), DQ_PD240_SOC-ODT48_VOH30_4266 (I/O), DQ_PD240_SOC-ODT60_VOH30_4266 (I/O), DQ_PD240_SOC-ODT80_VOH30_4266 (I/O), DQ_PD240_SOC-ODT120_VOH30_4266 (I/O), DQ_PD240_SOC-ODT240_VOH30_4266 (I/O), DQ_PD240_SOC-ODTDIS_VOH30_4266 (I/O), DQ_PD240_SOC-ODT80_VOH25_4266 (I/O), DQ_PD240_SOC-ODT120_VOH25_4266 (I/O), DQ_PD240_SOC-ODT240_VOH25_4266 (I/O), DQ_PD240_SOC-ODTDIS_VOH25_4266 (I/O), DQ_IN_ODTOFF_4266 (Input), DQ_IN_ODT40_4266 (Input), DQ_IN_ODT48_4266 (Input), DQ_IN_ODT60_4266 (Input), DQ_IN_ODT80_4266 (Input), DQ_IN_ODT120_4266 (Input), DQ_IN_ODT240_4266 (Input), DQS_PD40_SOC-ODT40_VOH30_4266 (I/O), DQS_PD40_SOC-ODT48_VOH30_4266 (I/O), DQS_PD40_SOC-ODT60_VOH30_4266 (I/O), DQS_PD40_SOC-ODT80_VOH30_4266 (I/O), DQS_PD40_SOC-ODT120_VOH30_4266 (I/O), DQS_PD40_SOC-ODT240_VOH30_4266 (I/O), DQS_PD40_SOC-ODTDIS_VOH30_4266 (I/O)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
